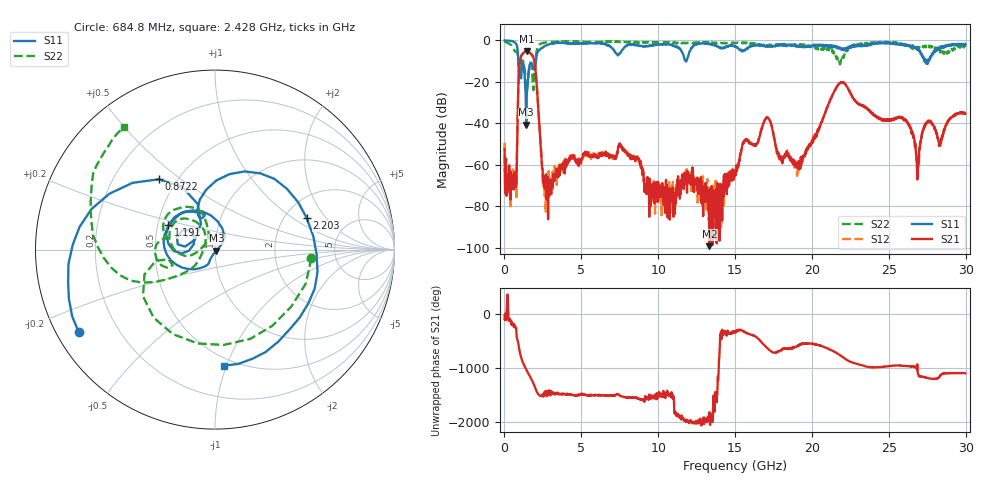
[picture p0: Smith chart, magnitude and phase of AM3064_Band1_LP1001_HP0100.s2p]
# Hz S DB R 50.0
!freq dBS11 angS11 dBS21 angS21 dBS12 angS12 dBS22 angS22
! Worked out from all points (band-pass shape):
!   1600 points, 10 MHz to 29.98 GHz, reference 50 ohm
!   highest |S21| = -5.06 dB at 1.435 GHz (marker M1); lowest = -99.2 dB at 13.34 GHz (marker M2)
!   |S21| within 3 dB of the highest: 1.065 GHz to 1.867 GHz (802.7 MHz wide, 54.8 % of centre)
!   lowest |S11| = -40.7 dB at 1.416 GHz (marker M3), VSWR 1.02, Z = 50.7 - j0.56 ohm
!   |S11| at or under -10 dB: 902.1 MHz to 2.045 GHz (1.143 GHz wide, 77.6 % of centre); 27.39387 GHz to 27.45789 GHz (64.02 MHz wide, 0.233 % of centre); 27.48841 GHz to 27.56234 GHz (73.94 MHz wide, 0.269 % of centre)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
!   |S22| runs from -24.3 to -0.3 dB; largest |S21 - S12| = 0.0072
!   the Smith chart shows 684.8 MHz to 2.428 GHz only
!   S11 on the Smith chart (normalised r, x): 684.8 MHz: 0.06, -0.28; 872.2 MHz: 0.40, +0.42; 1.191 GHz: 0.57, +0.17; 2.203 GHz: 2.62, +1.30; 2.428 GHz: 0.44, -0.98
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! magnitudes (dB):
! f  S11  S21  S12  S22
! 10 MHz  0.0  -52.3  -49.4  -0.3
! 684.8 MHz  -1.0  -66.9  -66.1  -5.4
! 872.2 MHz  -6.0  -31.0  -30.9  -7.6
! 1.191 GHz  -10.7  -6.5  -6.4  -9.7
! 1.416 GHz  -40.7  -5.1  -5.0  -23.3
! 1.435 GHz  -31.0  -5.1  -5.0  -24.2
! 2.203 GHz  -5.3  -32.9  -32.8  -2.8
! 2.428 GHz  -3.8  -59.7  -59.1  -1.4
! 2.897 GHz  -1.9  -73.3  -71.0  -0.9
! 5.015 GHz  -1.4  -57.2  -57.4  -0.6
! 7.545 GHz  -5.9  -50.7  -51.2  -0.8
! 10 GHz  -2.0  -68.3  -73.8  -0.9
! 13.34 GHz  -1.5  -99.2  -71.2  -1.1
! 15 GHz  -3.0  -63.1  -64.5  -1.4
! 17.05 GHz  -2.9  -37.4  -37.4  -2.6
! 17.99 GHz  -2.4  -55.8  -56.2  -2.3
! 19.99 GHz  -2.8  -49.2  -48.8  -3.0
! 21.88 GHz  -4.0  -20.5  -20.3  -9.7
! 25 GHz  -1.0  -38.5  -38.6  -1.1
! 26.89 GHz  -4.0  -61.8  -66.7  -3.5
! 27.47 GHz  -9.6  -39.8  -39.6  -2.7
! 29.98 GHz  -1.8  -35.4  -35.0  -3.2
